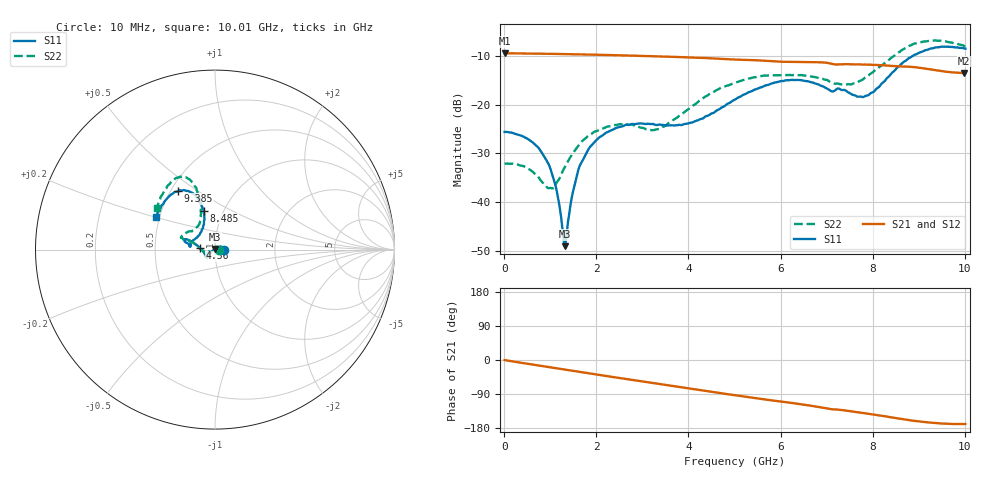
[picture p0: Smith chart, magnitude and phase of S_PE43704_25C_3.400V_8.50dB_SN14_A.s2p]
! Device ID: PE43704
! Dir: z:\PE43704\PE43704_Char_1_20130516\PE43704\AMB\3p400V\8p50dB
! Serial: 14
! Insertion: A
! Impedance: 50 ohm
! Temp: Amb
! VDD: 3.400V
! Attenuation Step: 8.50dB
! IDD: 1.140658e-01mA
#  Hz  S  RI  R  50
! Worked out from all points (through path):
!   401 points, 10 MHz to 10.01 GHz, reference 50 ohm
!   highest |S21| = -9.48 dB at 10 MHz (marker M1); lowest = -13.5 dB at 9.985 GHz (marker M2)
!   group delay of S21, straight-line fit = 48.7 ps
!   lowest |S11| = -49.0 dB at 1.31 GHz (marker M3), VSWR 1.01, Z = 49.9 + j0.322 ohm
!   |S11| at or under -10 dB: start of sweep to 8.873 GHz
!   |S22| runs from -37.2 to -6.9 dB; largest |S21 - S12| = 0.0027
!   S11 on the Smith chart (normalised r, x): 10 MHz: 1.11, +0.00; 4.56 GHz: 0.85, +0.01; 8.485 GHz: 0.81, +0.37; 9.385 GHz: 0.55, +0.42; 10.01 GHz: 0.48, +0.20
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1e7  0.0524 0.000186  0.3357 -0.00127  0.3358 -0.00123  0.0247 0.000267
5.35e8  0.041 0.0151  0.3276 -0.0603  0.3275 -0.0602  0.0154 0.0155
9.1e8  0.0226 0.0152  0.3158 -0.1  0.3157 -0.0999  -0.000732 0.0146
1.11e9  0.0108 0.0106  0.3077 -0.1206  0.3078 -0.1204  -0.0117 0.00916
1.31e9  -0.00145 0.00323  0.2976 -0.1402  0.2978 -0.1401  -0.0225 0.00116
1.36e9  -0.00472 0.00103  0.2952 -0.1449  0.2951 -0.1448  -0.025 -0.000923
1.51e9  -0.0125 -0.00574  0.2866 -0.1588  0.2867 -0.1587  -0.0315 -0.00829
1.685e9  -0.0215 -0.0143  0.2761 -0.1746  0.2761 -0.1744  -0.0382 -0.0171
1.91e9  -0.0303 -0.0242  0.261 -0.1932  0.2611 -0.1932  -0.0428 -0.027
2.26e9  -0.0379 -0.0366  0.2352 -0.2198  0.2353 -0.2196  -0.0474 -0.0364
3.36e9  -0.0475 -0.0403  0.1399 -0.2781  0.1402 -0.2779  -0.0533 -0.0179
4.56e9  -0.0827 0.00805  0.0247 -0.2953  0.0251 -0.2954  -0.1285 0.0433
5.01e9  -0.1084 0.0297  -0.0145 -0.2891  -0.0142 -0.2894  -0.1597 0.0499
5.96e9  -0.1615 0.0582  -0.089 -0.261  -0.0882 -0.2612  -0.1881 0.0672
6.685e9  -0.1639 0.0408  -0.1414 -0.2325  -0.1412 -0.2321  -0.1744 0.0836
7.36e9  -0.1357 0.0388  -0.1748 -0.1912  -0.1747 -0.1909  -0.113 0.1161
7.76e9  -0.0913 0.078  -0.1956 -0.167  -0.1954 -0.1675  -0.083 0.1573
8.36e9  -0.0599 0.1872  -0.2174 -0.123  -0.2169 -0.1245  -0.0856 0.2771
8.485e9  -0.0639 0.2167  -0.2213 -0.1122  -0.2199 -0.1134  -0.0929 0.3086
9.385e9  -0.205 0.3268  -0.218 -0.0517  -0.2187 -0.0506  -0.2256 0.3911
9.985e9  -0.3237 0.1895  -0.2064 -0.04  -0.2074 -0.0405  -0.3194 0.2377
1.001e10  -0.3286 0.1795  -0.2072 -0.0408  -0.2088 -0.0411  -0.3229 0.2296
